FUNCTION "RULLI_GUIDA_INF" : VOID
TITLE =GUIDA LAMIERA INGRESSO FEEDER
AUTHOR : Davi
FAMILY : linea
NAME : feeder
VERSION : 0.1

BEGIN
NETWORK
TITLE =COMANDO MANUALE MOTORE FRONTE
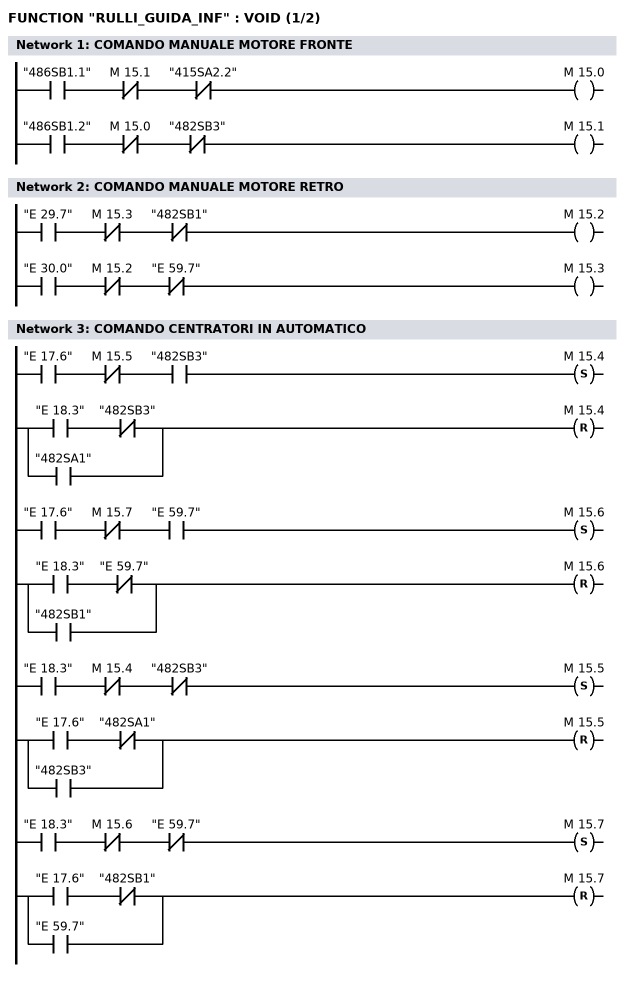
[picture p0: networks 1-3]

// Motore avanti
      U     "486SB1.1";
      UN    M     15.1;
      UN    "415SA2.2";
      =     M     15.0;
// Motore indietro
      U     "486SB1.2";
      UN    M     15.0;
      UN    "482SB3";
      =     M     15.1;

NETWORK
TITLE =COMANDO MANUALE MOTORE RETRO

// Motore avanti
      U     "E      29.7";
      UN    M     15.3;
      UN    "482SB1";
      =     M     15.2;
// Motore indietro
      U     "E      30.0";
      UN    M     15.2;
      UN    "E      59.7";
      =     M     15.3;


NETWORK
TITLE =COMANDO CENTRATORI IN AUTOMATICO

// Motori avanti
      U     "E      17.6";
      UN    M     15.5;
      U     "482SB3";
      S     M     15.4;

      U     "E      18.3";
      UN    "482SB3";
      O     "482SA1";
      R     M     15.4;

      U     "E      17.6";
      UN    M     15.7;
      U     "E      59.7";
      S     M     15.6;

      U     "E      18.3";
      UN    "E      59.7";
      O     "482SB1";
      R     M     15.6;

// Motori indietro
      U     "E      18.3";
      UN    M     15.4;
      UN    "482SB3";
      S     M     15.5;

      U     "E      17.6";
      UN    "482SA1";
      O     "482SB3";
      R     M     15.5;

      U     "E      18.3";
      UN    M     15.6;
      UN    "E      59.7";
      S     M     15.7;

      U     "E      17.6";
      UN    "482SB1";
      O     "E      59.7";
      R     M     15.7;

NETWORK
TITLE =COMANDO MOTORI
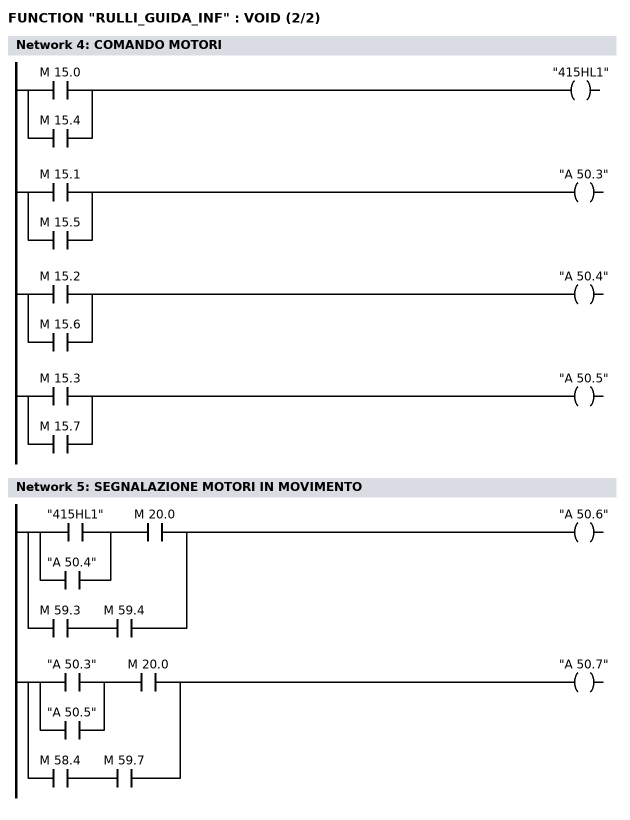
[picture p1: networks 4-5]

// Fronte avanti
      O     M     15.0;
      O     M     15.4;
      =     "415HL1";
// Fronte indietro
      O     M     15.1;
      O     M     15.5;
      =     "A      50.3";
// Retro avanti
      O     M     15.2;
      O     M     15.6;
      =     "A      50.4";
// Retro indietro
      O     M     15.3;
      O     M     15.7;
      =     "A      50.5";

NETWORK
TITLE =SEGNALAZIONE MOTORI IN MOVIMENTO

      U(    ;
      O     "415HL1";
      O     "A      50.4";
      )     ;
      U     M     20.0;
      O(    ;
      U     M     59.3;
      U     M     59.4;
      )     ;
      =     "A      50.6";

      U(    ;
      O     "A      50.3";
      O     "A      50.5";
      )     ;
      U     M     20.0;
      O(    ;
      U     M     58.4;
      U     M     59.7;
      )     ;
      =     "A      50.7";

NETWORK
TITLE =ALLARME TERMICI



END_FUNCTION

